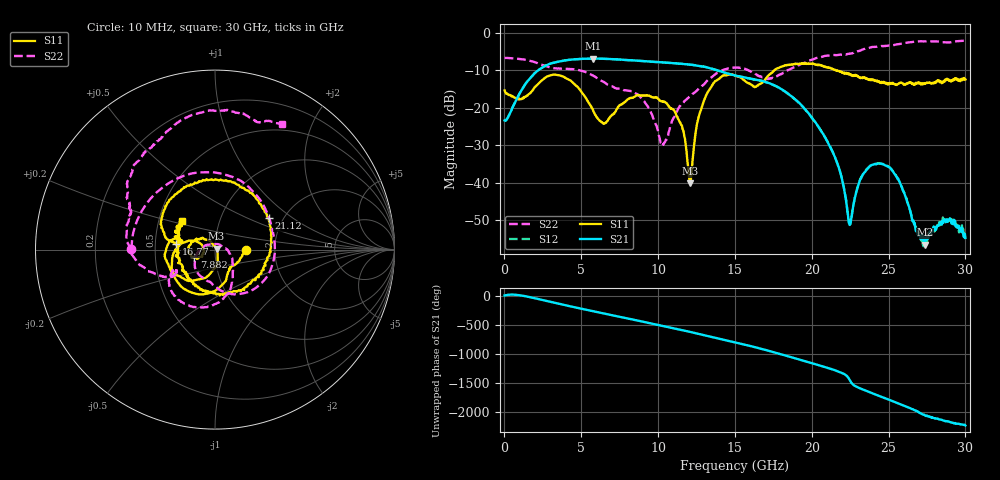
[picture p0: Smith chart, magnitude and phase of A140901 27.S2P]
!  2-Port S-parameters saved by WinCal
! VAR MeasName=S-Parameters (CALIBRATED_DATA) read from VNA (N5244A)
! VAR MeasDate=11/3/2014 9:29:02 AM
! VAR NAME=A140901 27
! VAR FILENAME=A140901 27.S2P
! VAR DATE=11/3/2014 9:29:02 AM
! VAR PHYS_PORTS=1,2
# Hz S RI R 50
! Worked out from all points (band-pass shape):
!   801 points, 10 MHz to 30 GHz, reference 50 ohm
!   highest |S21| = -6.82 dB at 5.783 GHz (marker M1); lowest = -56.5 dB at 27.38 GHz (marker M2)
!   |S21| within 3 dB of the highest: 2.241 GHz to 13.76 GHz (11.52 GHz wide, 144 % of centre)
!   lowest |S11| = -40.1 dB at 12.08 GHz (marker M3), VSWR 1.02, Z = 50.9 + j0.467 ohm
!   |S11| at or under -10 dB: start of sweep to 17.56 GHz; 21.60188 GHz to 21.60325 GHz (1.367 MHz wide, 0.00633 % of centre); 21.65 GHz to end of sweep
!   |S22| runs from -30.1 to -2.0 dB; largest |S21 - S12| = 0.0028
!   S11 on the Smith chart (normalised r, x): 10 MHz: 1.41, -0.01; 7.882 GHz: 0.79, -0.07; 16.77 GHz: 0.65, +0.04; 21.12 GHz: 1.68, +0.67; 30 GHz: 0.66, +0.22
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1e7  0.1714 -0.00473  0.0683 0.000168  0.0676 0.000652  -0.4653 0.00421
1.35955e9  0.0755 -0.1195  0.2037 -0.0449  0.2039 -0.0449  -0.092 0.43
2.971512e9  -0.128 -0.2399  -0.1204 -0.3701  -0.1201 -0.37  0.3032 0.1704
5.033325e9  -0.1551 0.0462  -0.3019 0.3365  -0.3013 0.3368  0.2322 -0.2099
5.783075e9  -0.0839 0.0348  0.00216 0.456  0.00206 0.4551  0.1033 -0.2488
7.882375e9  -0.1149 -0.0428  0.3912 -0.1943  0.3909 -0.1935  -0.061 -0.1611
1.001916e10  -0.1243 0.0448  -0.3345 -0.2362  -0.334 -0.2363  -0.0388 0.0277
1.039404e10  -0.1046 0.0589  -0.3923 -0.0987  -0.3914 -0.099  0.0123 0.0323
1.148118e10  -0.0316 0.0513  -0.2569 0.2917  -0.257 0.2917  0.0962 -0.0529
1.208098e10  0.00872 0.00459  -0.0375 0.3772  -0.0376 0.3771  0.0991 -0.1035
1.313062e10  -0.0354 -0.1441  0.3 0.1807  0.3013 0.1797  0.0894 -0.2057
1.5005e10  -0.2717 0.00408  0.0316 -0.2696  0.0296 -0.268  -0.1762 -0.2975
1.676691e10  -0.2147 0.0298  -0.2193 0.0696  -0.218 0.0685  -0.2288 -0.1165
1.849134e10  -0.2406 0.2905  0.1254 0.0878  0.1246 0.0872  -0.2828 -0.153
2.002832e10  0.0873 0.3809  0.00888 -0.0726  0.00991 -0.0725  -0.4359 -0.0654
2.111546e10  0.2983 0.176  -0.032 -0.00678  -0.0323 -0.00728  -0.4926 0.0923
2.246501e10  0.2367 -0.1505  0.00273 -0.000289  0.00284 -0.000204  -0.4793 0.2318
2.34022e10  0.0321 -0.2484  -0.0136 0.000292  -0.0137 4.64e-05  -0.4918 0.3665
2.501416e10  -0.1626 -0.1266  0.016 0.00403  0.0159 0.00398  -0.3316 0.5951
2.737588e10  -0.2131 0.0283  -0.000359 0.00146  -0.000669 0.00169  0.036 0.7746
2.891286e10  -0.2192 0.0975  0.00323 -0.000124  0.00302 -0.000318  0.2397 0.7093
3e10  -0.1821 0.1573  0.000671 -0.00171  0.000689 -0.00202  0.3752 0.6997
